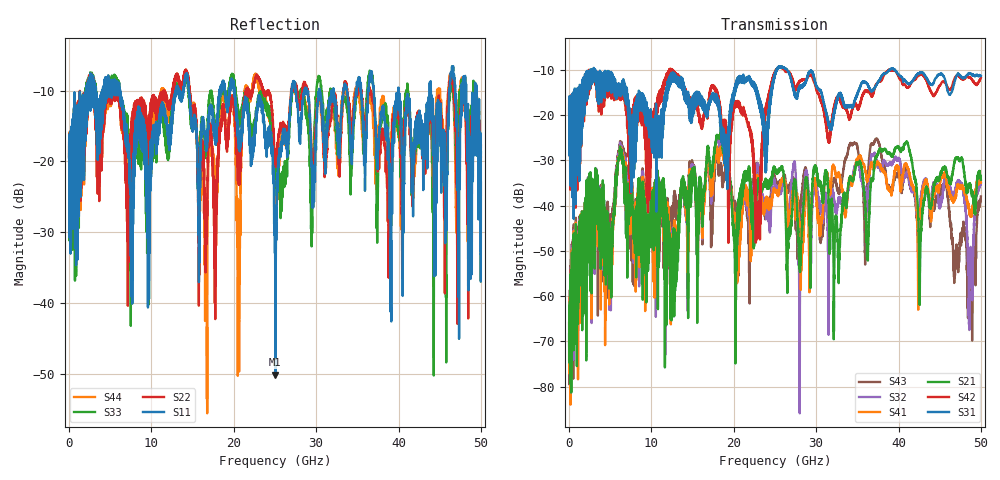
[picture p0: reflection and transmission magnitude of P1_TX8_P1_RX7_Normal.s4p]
!Keysight Technologies,N5225B,MY57041031,A.13.20.10
!Date: Friday, May 31, 2019 11:24:40
!Correction: S11(Full 4 Port(1,2,3,4))
!S12(Full 4 Port(1,2,3,4))
!S13(Full 4 Port(1,2,3,4))
!S14(Full 4 Port(1,2,3,4))
!S21(Full 4 Port(1,2,3,4))
!S22(Full 4 Port(1,2,3,4))
!S23(Full 4 Port(1,2,3,4))
!S24(Full 4 Port(1,2,3,4))
!S31(Full 4 Port(1,2,3,4))
!S32(Full 4 Port(1,2,3,4))
!S33(Full 4 Port(1,2,3,4))
!S34(Full 4 Port(1,2,3,4))
!S41(Full 4 Port(1,2,3,4))
!S42(Full 4 Port(1,2,3,4))
!S43(Full 4 Port(1,2,3,4))
!S44(Full 4 Port(1,2,3,4))
!S4P File: Measurements: <S11,S12,S13,S14>,
!<S21,S22,S23,S24>,
!<S31,S32,S33,S34>,
!<S41,S42,S43,S44>:
# Hz S  dB  R 50.0
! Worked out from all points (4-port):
!   5000 points, 10 MHz to 50 GHz, reference 50 ohm
!   strongest paths, dB at 10 MHz, 12.51 GHz, 25.01 GHz, 37.51 GHz, 50 GHz:
!     S31: -19.6, -10.9, -11.1, -12.7, -11.3
!     S42: -19.6, -10.0, -10.6, -12.7, -11.8
!     S21: -68.4, -53.4, -31.9, -28.7, -34.3
!     S41: -74.1, -49.7, -36.7, -30.5, -34.8
!     S32: -70.4, -46.8, -35.3, -31.3, -35.0
!     S43: -65.9, -43.3, -33.9, -25.8, -38.0
!   lowest |S11| = -50.1 dB at 25.05 GHz (marker M1), VSWR 1.01, Z = 49.7 - j0.0503 ohm
!   |S11| at or under -10 dB: 6.191 GHz to 12.97 GHz (6.783 GHz wide, 70.8 % of centre); 20.1 GHz to 27.04 GHz (6.942 GHz wide, 29.5 % of centre); 40 GHz to 43.76 GHz (3.767 GHz wide, 8.99 % of centre)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
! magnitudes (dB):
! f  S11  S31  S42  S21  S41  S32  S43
! 10 MHz  -19.5  -19.6  -19.6  -68.4  -74.1  -70.4  -65.9
! 6.24 GHz  -10.8  -13.6  -14.1  -27.5  -27.5  -26.9  -26.4
! 12.57 GHz  -13.8  -10.7  -10.4  -57.2  -46.2  -47.1  -40.1
! 16.62 GHz  -17.6  -18.3  -18.4  -31.6  -32.9  -32.2  -33.3
! 22.93 GHz  -11.7  -15.9  -39.6  -36.0  -34.9  -31.3  -31.8
! 25.05 GHz  -50.1  -10.5  -10.4  -32.4  -36.9  -35.8  -34.3
! 50 GHz  -23.0  -11.3  -11.8  -34.3  -34.8  -35.0  -38.0
